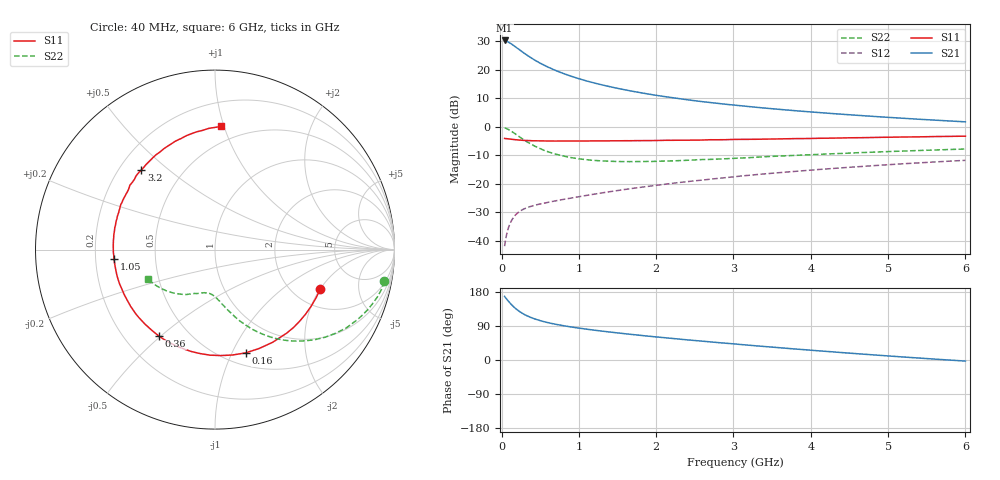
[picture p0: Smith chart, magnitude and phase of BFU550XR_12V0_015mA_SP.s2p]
! Filename:  P:\Prog\Test\Noise\ATS_data\Testdata_Net\03 Spar\BFU550XR_APG2013_45_C05_12p0V_015mA_SP_CM01_D.s2p
! Date/Time: Tue 06/Aug/2013 14:38:19
! BFU550XR_APG2013_45_C05_12p0V_1to35mA_SP_CM01_Bias6_R.s2p
! MDIF S-parameter v. bias file
! BFU550XR_APG2013_45_C05_12p0V_1to35mA_SP_CM01
! Date/time Fri Aug 02 14:58:10 2013
! VAR V_out= 12.0010
! VAR I_out= 14.9950
! VAR V_in= 0.7897
! VAR I_in= 0.1431
! Device data file deembeded for feedlines and parallel
! Original file: \03 Spar\BFU550XR_APG2013_45_C05_12p0V_015mA_SP_CM01_R.s2p
! Feed-files: PR006V01_02082013_Feed1.s2p, PR006V01_02082013_Feed2.s2p
! Parallel-file: PR006V01_02082013_Par.s2p
# MHz S MA R 50
!  Freq-MHz  S11-mag  S11-arg  S21-mag  S21-arg  S12-mag  S12-arg  S22-mag  S22-arg
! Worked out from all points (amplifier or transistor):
!   98 points, 40 MHz to 6 GHz, reference 50 ohm
!   highest |S21| = 30.4 dB at 40 MHz (marker M1)
!   |S21| within 3 dB of that: start of sweep to 219.1 MHz
!   unconditionally stable (mu >= 1): 1.763 GHz to 3.726 GHz
!   at 300 MHz: K = 0.36, MSG = 27.2 dB, |S12| = -28.7 dB
!   at 1.6 GHz: K = 0.98, MSG = 17.5 dB, |S12| = -22.0 dB
!   at 6 GHz: K = 0.88, MSG = 6.8 dB, |S12| = -11.8 dB
!   S11 on the Smith chart (normalised r, x): 40 MHz: 2.78, -2.01; 160 MHz: 0.63, -1.13; 360 MHz: 0.34, -0.50; 1.05 GHz: 0.28, -0.04; 3.2 GHz: 0.29, +0.41; 6 GHz: 0.38, +0.98
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40  0.6268 -20.5  32.98 167.9  0.008024 77.7  0.9608 -10.7
50  0.6239 -25.5  32.75 164.7  0.009933 76.3  0.9533 -13.6
100  0.6133 -49.4  30.2 152.6  0.01848 68.1  0.8843 -26.2
120  0.6083 -58.1  29.13 148.0  0.02135 64.9  0.8526 -30.7
160  0.6002 -73.4  26.68 140.0  0.02625 59.6  0.7842 -38.5
180  0.5953 -80.5  25.51 136.3  0.0283 57.3  0.7496 -42.0
220  0.5888 -92.7  23.3 129.8  0.03169 53.8  0.6865 -48.0
260  0.5829 -103.0  21.24 124.4  0.03441 50.9  0.6293 -53.1
300  0.5788 -112.0  19.43 119.7  0.03663 48.8  0.5796 -57.4
360  0.5741 -122.7  17.1 114.0  0.03937 46.7  0.5172 -62.6
400  0.5705 -128.9  15.79 110.6  0.04087 45.8  0.482 -65.6
460  0.5685 -136.4  14.11 106.5  0.04299 45.0  0.439 -69.1
600  0.5647 -150.0  11.26 98.7  0.04721 44.8  0.3661 -75.7
800  0.5649 -163.0  8.677 90.6  0.05323 46.0  0.3082 -82.3
1050  0.5653 -174.6  6.711 82.8  0.06091 48.1  0.2698 -88.3
1500  0.5696 170.4  4.759 71.5  0.07614 50.6  0.2469 -96.7
2050  0.5775 156.8  3.501 60.0  0.0958 51.6  0.2497 -105.2
3100  0.6038 134.7  2.348 40.8  0.137 49.5  0.2837 -119.3
3200  0.6043 132.7  2.275 39.0  0.1411 49.0  0.2878 -120.4
4100  0.6302 117.0  1.788 24.3  0.1782 44.1  0.3287 -132.2
5200  0.664 99.0  1.416 7.9  0.2252 36.3  0.3763 -146.2
6000  0.6873 87.1  1.226 -2.9  0.2582 29.8  0.4085 -156.4
